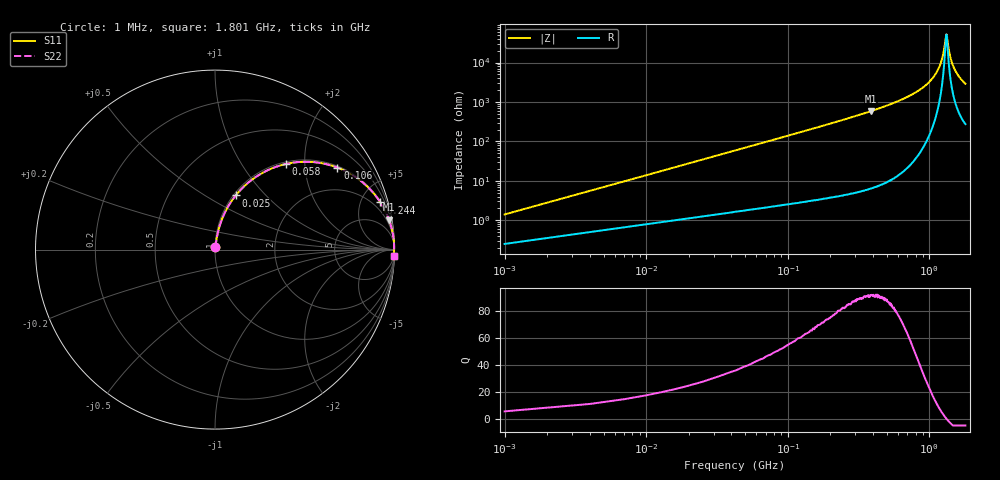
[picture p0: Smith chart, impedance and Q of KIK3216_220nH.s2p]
!version-2
!date-01.2022
!Series
# MHz S RI R 50
!Freq ReS11 ImS11 ReS21 ImS21 ReS12 ImS12 ReS22 ImS22
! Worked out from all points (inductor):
!   601 points, 1 MHz to 1.801 GHz, reference 50 ohm
!   read as one part in series: L = 220 nH near 10 MHz
!   highest Q = 92.1 at 385 MHz (marker M1), where L = 240 nH
!   self-resonance near 1.321 GHz
!   S11 on the Smith chart (normalised r, x): 1 MHz: 1.00, +0.03; 25 MHz: 1.03, +0.69; 58 MHz: 1.04, +1.61; 106 MHz: 1.05, +2.95; 244 MHz: 1.08, +6.98; 1.801 GHz: 7, -58
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1  0.00268 0.0138  0.9973 -0.0138  0.9973 -0.0138  0.00268 0.0138
13  0.0394 0.1711  0.9606 -0.1711  0.9606 -0.1711  0.0394 0.1711
19  0.0733 0.2408  0.9266 -0.2408  0.9266 -0.2408  0.0733 0.2408
25  0.1155 0.302  0.8845 -0.302  0.8845 -0.302  0.1155 0.302
40  0.2409 0.4136  0.7591 -0.4136  0.7591 -0.4136  0.2409 0.4136
58  0.3948 0.4771  0.6052 -0.4771  0.6052 -0.4771  0.3948 0.4771
106  0.6821 0.4569  0.3179 -0.4569  0.3179 -0.4569  0.6821 0.4569
163  0.8361 0.3631  0.1639 -0.3631  0.1639 -0.3631  0.8361 0.3631
244  0.9215 0.263  0.0785 -0.263  0.0785 -0.263  0.9215 0.263
301  0.9484 0.2156  0.0516 -0.2156  0.0516 -0.2156  0.9484 0.2156
385  0.9696 0.1664  0.0304 -0.1664  0.0304 -0.1664  0.9696 0.1664
601  0.9898 0.0944  0.0102 -0.0944  0.0102 -0.0944  0.9898 0.0944
901  0.9969 0.0428  0.00309 -0.0428  0.00309 -0.0428  0.9969 0.0428
1084  0.998 0.0219  0.00196 -0.0219  0.00196 -0.0219  0.998 0.0219
1201  0.9982 0.0106  0.00179 -0.0106  0.00179 -0.0106  0.9982 0.0106
1255  0.9982 0.00576  0.00182 -0.00576  0.00182 -0.00576  0.9982 0.00576
1309  0.9981 0.00117  0.0019 -0.00117  0.0019 -0.00117  0.9981 0.00117
1324  0.9981 -6.92e-05  0.00193 6.92e-05  0.00193 6.92e-05  0.9981 -6.92e-05
1405  0.9978 -0.00653  0.00216 0.00653  0.00216 0.00653  0.9978 -0.00653
1501  0.9975 -0.0137  0.00254 0.0137  0.00254 0.0137  0.9975 -0.0137
1627  0.9968 -0.0226  0.00321 0.0226  0.00321 0.0226  0.9968 -0.0226
1801  0.9956 -0.0339  0.00438 0.0339  0.00438 0.0339  0.9956 -0.0339
